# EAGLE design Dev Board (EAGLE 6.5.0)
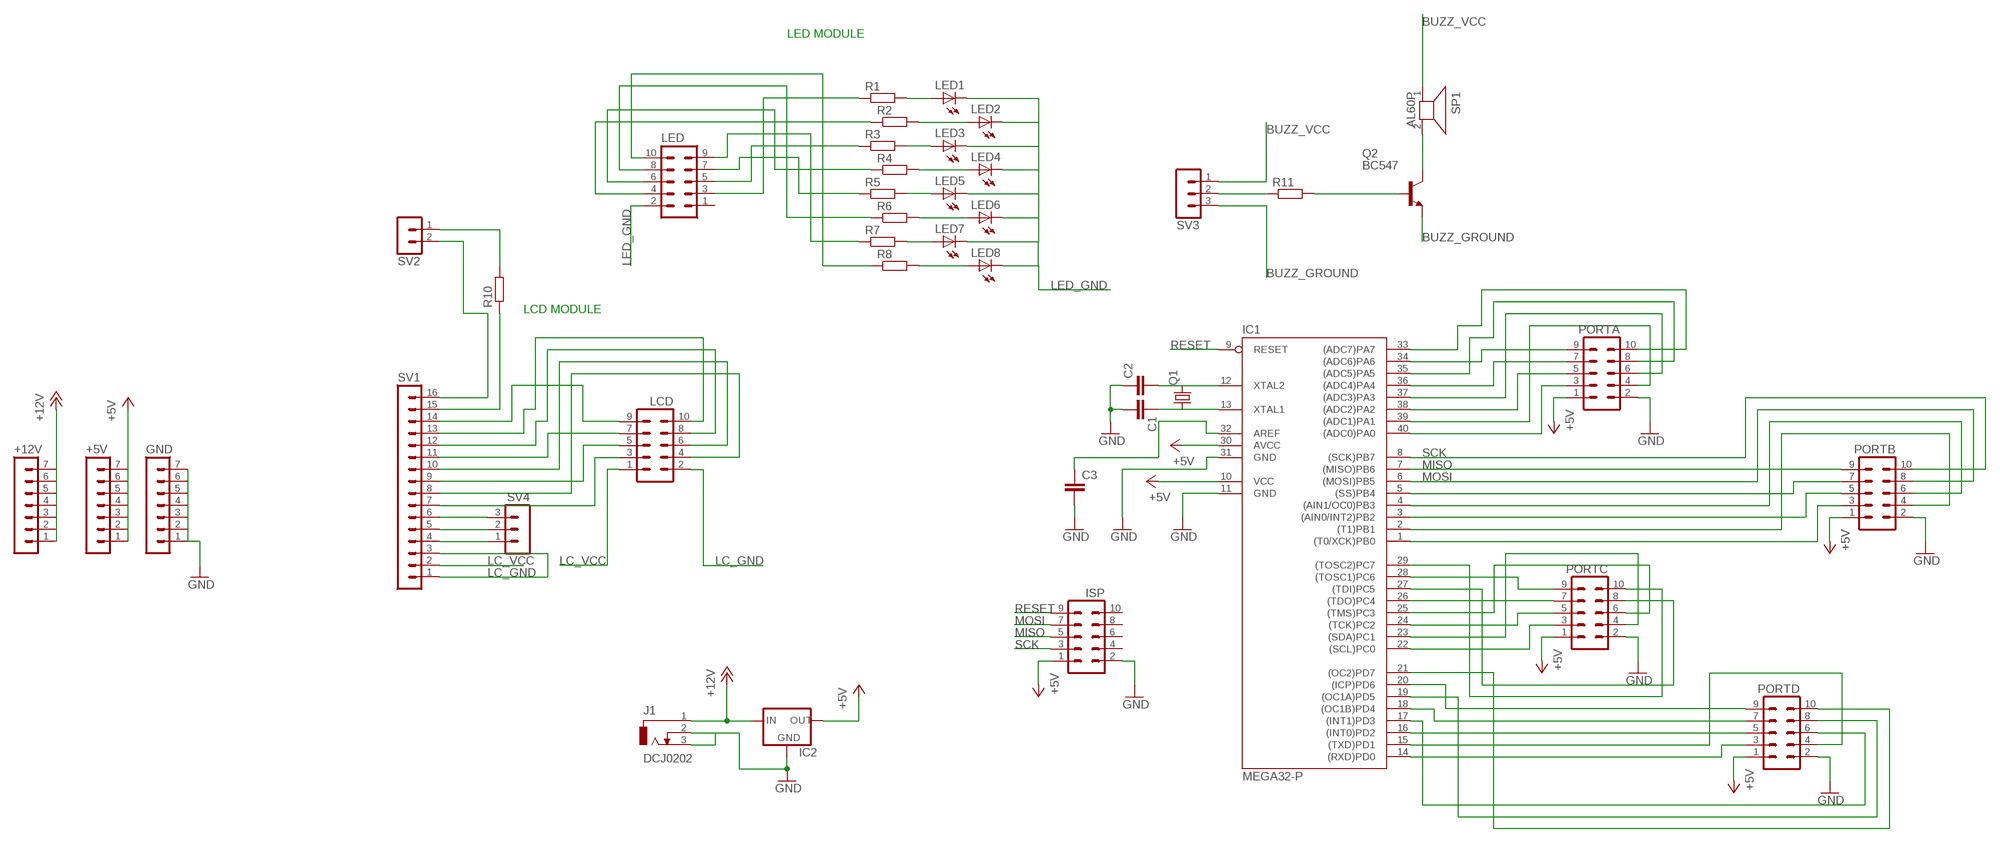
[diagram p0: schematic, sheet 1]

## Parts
+5V  MA07-1  [MA07-1]
+12V  MA07-1  [MA07-1]
C1  C-EU025-024X044  [C025-024X044]
C2  C-EU025-024X044  [C025-024X044]
C3  C-EU025-024X044  [C025-024X044]
GND  MA07-1  [MA07-1]
IC1  MEGA32-P  [DIL40]
IC2  78XXL  [78XXL]
ISP  MA05-2  [MA05-2]
J1  DCJ0202  [DCJ0202]
LCD  MA05-2  [MA05-2]
LED  MA05-2  [MA05-2]
LED1  LED3MM  [LED3MM]
LED2  LED3MM  [LED3MM]
LED3  LED3MM  [LED3MM]
LED4  LED3MM  [LED3MM]
LED5  LED3MM  [LED3MM]
LED6  LED3MM  [LED3MM]
LED7  LED3MM  [LED3MM]
LED8  LED3MM  [LED3MM]
PORTA  MA05-2  [MA05-2]
PORTB  MA05-2  [MA05-2]
PORTC  MA05-2  [MA05-2]
PORTD  MA05-2  [MA05-2]
Q1  CRYSTALHC49S  [HC49/S]
Q2  BC547  [TO92]
R1  R-EU_0207/10  [0207/10]
R2  R-EU_0207/10  [0207/10]
R3  R-EU_0207/10  [0207/10]
R4  R-EU_0207/10  [0207/10]
R5  R-EU_0207/10  [0207/10]
R6  R-EU_0207/10  [0207/10]
R7  R-EU_0207/10  [0207/10]
R8  R-EU_0207/10  [0207/10]
R10  R-EU_0207/10  [0207/10]
R11  R-EU_0207/10  [0207/10]
SP1  AL60P  [AL60P]
SV1  MA13-1  [MA13-1]
SV2  MA03-1  [MA03-1]
SV3  MA03-1  [MA03-1]
SV4  MA03-1  [MA03-1]

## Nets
+5V: +5V.1 +5V.2 +5V.3 +5V.4 +5V.5 +5V.6 +5V.7 IC1.10(VCC) IC1.30(AVCC) IC2.OUT ISP.1 PORTA.1 PORTB.1 PORTC.1 PORTD.1
+12V: +12V.1 +12V.2 +12V.3 +12V.4 +12V.5 +12V.6 +12V.7 IC2.IN J1.1
BUZZ_GROUND: Q2.1(E) SV3.3
BUZZ_VCC: SP1.1 SV3.1
GND: C1.2 C2.1 C3.2 GND.1 GND.2 GND.3 GND.4 GND.5 GND.6 GND.7 IC1.11(GND) IC1.31(GND) IC2.GND ISP.2 J1.2 J1.3 PORTA.2 PORTB.2 PORTC.2 PORTD.2
LC_GND: LCD.2 SV1.1 SV1.3
LC_VCC: LCD.1 SV1.2
LCD_GND: SV1.16 SV2.2
LED_GND: LED1.K(C) LED2.K(C) LED3.K(C) LED4.K(C) LED5.K(C) LED6.K(C) LED7.K(C) LED8.K(C) LED.2
MISO: IC1.7((MISO)PB6) ISP.5 PORTB.9
MOSI: IC1.6((MOSI)PB5) ISP.7 PORTB.8
N$1: LED1.A R1.2
N$2: LED2.A R2.2
N$3: LED3.A R3.2
N$4: LED4.A R4.2
N$5: LED5.A R5.2
N$6: LED6.A R6.2
N$7: LED7.A R7.2
N$8: LED8.A R8.2
N$9: IC1.40((ADC0)PA0) PORTA.3
N$10: IC1.38((ADC2)PA2) PORTA.5
N$11: IC1.36((ADC4)PA4) PORTA.7
N$12: IC1.34((ADC6)PA6) PORTA.9
N$13: IC1.39((ADC1)PA1) PORTA.4
N$14: IC1.37((ADC3)PA3) PORTA.6
N$15: IC1.35((ADC5)PA5) PORTA.8
N$17: LED.3 R1.1
N$18: LED.4 R2.1
N$19: LED.5 R3.1
N$20: LED.6 R4.1
N$21: LED.7 R5.1
N$22: LED.8 R6.1
N$23: LED.9 R7.1
N$24: LED.10 R8.1
N$25: IC1.33((ADC7)PA7) PORTA.10
N$26: IC1.1((T0/XCK)PB0) PORTB.3
N$27: IC1.3((AIN0/INT2)PB2) PORTB.5
N$28: IC1.5((SS)PB4) PORTB.7
N$30: IC1.2((T1)PB1) PORTB.4
N$31: IC1.4((AIN1/OC0)PB3) PORTB.6
N$32: R10.1 SV1.15
N$33: Q2.2(B) R11.2
N$34: IC1.22((SCL)PC0) PORTC.3
N$35: IC1.24((TCK)PC2) PORTC.5
N$36: IC1.26((TDO)PC4) PORTC.7
N$37: IC1.28((TOSC1)PC6) PORTC.9
N$38: IC1.23((SDA)PC1) PORTC.4
N$39: IC1.25((TMS)PC3) PORTC.6
N$40: IC1.27((TDI)PC5) PORTC.8
N$41: IC1.29((TOSC2)PC7) PORTC.10
N$42: IC1.14((RXD)PD0) PORTD.3
N$43: IC1.16((INT0)PD2) PORTD.5
N$44: IC1.18((OC1B)PD4) PORTD.7
N$45: IC1.20((ICP)PD6) PORTD.9
N$46: IC1.15((TXD)PD1) PORTD.4
N$47: IC1.17((INT1)PD3) PORTD.6
N$48: IC1.19((OC1A)PD5) PORTD.8
N$49: IC1.21((OC2)PD7) PORTD.10
N$50: C2.2 IC1.12(XTAL2) Q1.2
N$51: C1.1 IC1.13(XTAL1) Q1.1
N$52: SV1.4 SV4.1
N$53: LCD.3 SV1.7
N$54: SV1.5 SV4.2
N$55: SV1.6 SV4.3
N$56: LCD.5 SV1.9
N$57: LCD.7 SV1.11
N$58: LCD.9 SV1.14
N$59: LCD.4 SV1.8
N$60: LCD.6 SV1.10
N$61: LCD.8 SV1.12
N$62: LCD.10 SV1.13
N$63: R10.2 SV2.1
N$64: C3.1 IC1.32(AREF)
N$65: Q2.3(C) SP1.2
N$68: R11.1 SV3.2
RESET: IC1.9(RESET) ISP.9
SCK: IC1.8((SCK)PB7) ISP.3 PORTB.10
Unconnected: ISP.4 ISP.6 ISP.8 ISP.10 LED.1

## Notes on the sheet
- LED MODULE
- LCD MODULE

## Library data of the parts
+5V +12V GND = con-lstb:MA07-1: PIN HEADER; OC_FARNELL: unknown; OC_NEWARK: unknown
C1-C3 = rcl:C-EU: CAPACITOR, European symbol
IC1 = atmel:MEGA32-P: MICROCONTROLLER 32 Kbytes FLASH 2 Kbytes SRAM 1 Kbytes EEPROM USART 8-channel 10 bit ADC Source: www.atmel.com .. doc2503.pdf; MPN: ATMEGA32-16PU; OC_FARNELL: 1661729; OC_NEWARK: 51P1794
IC2 = v-reg:78XXL: VOLTAGE REGULATOR
ISP LCD LED PORTA PORTB PORTC PORTD = con-lstb:MA05-2: PIN HEADER; OC_FARNELL: unknown; OC_NEWARK: unknown
J1 = con-jack:DCJ0202: DC POWER JACK Source: DCJ0202.pdf; OC_FARNELL: unknown; OC_NEWARK: unknown
LED1-LED8 = led:LED: LED
Q1 = crystal:CRYSTAL: CRYSTAL; OC_FARNELL: 1667008; OC_NEWARK: unknown
Q2 = transistor-npn:BC547*: NPN Transistor
R1-R8 R10 R11 = rcl:R-EU_: RESISTOR, European symbol
SP1 = buzzer:AL60P: SPEAKER; OC_FARNELL: unknown; OC_NEWARK: unknown
SV1 = con-lstb-modified:MA13-1: PIN HEADER; OC_FARNELL: unknown; OC_NEWARK: unknown
SV2 = con-lstb-modified:MA03-1: PIN HEADER; OC_FARNELL: unknown; OC_NEWARK: unknown
SV3 SV4 = con-lstb:MA03-1: PIN HEADER; OC_FARNELL: unknown; OC_NEWARK: unknown

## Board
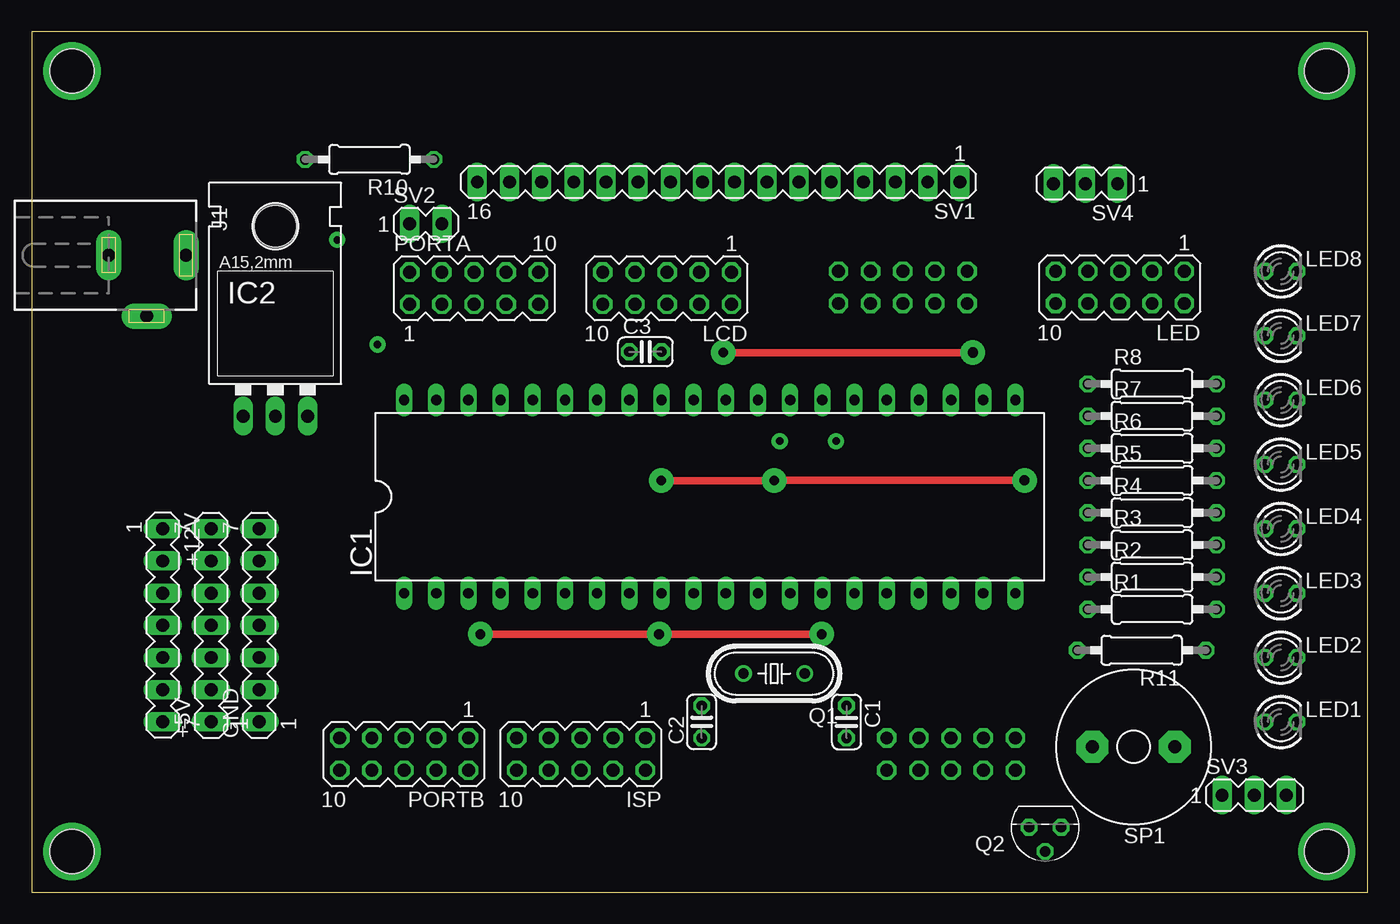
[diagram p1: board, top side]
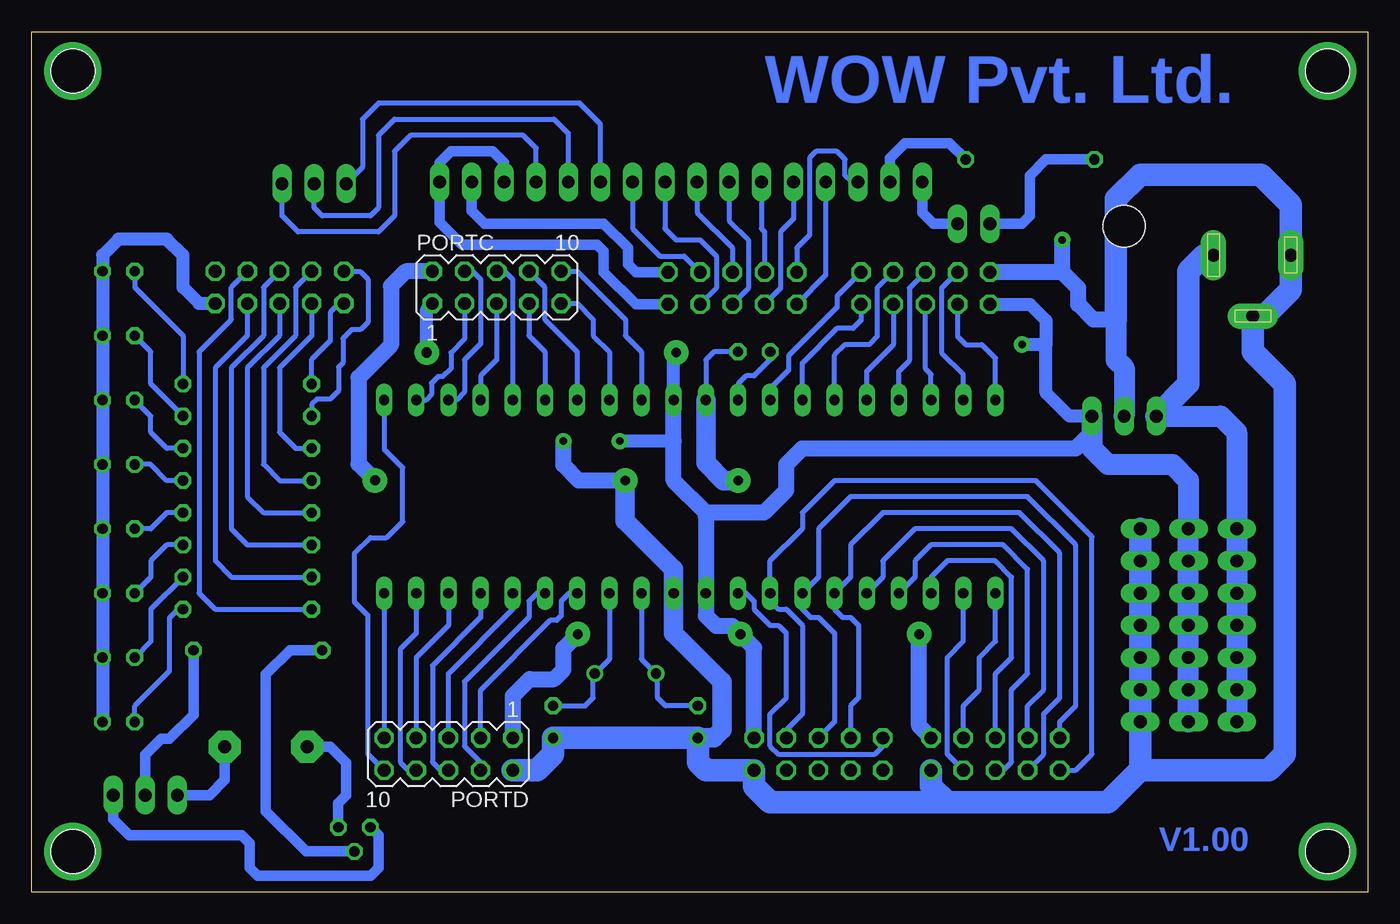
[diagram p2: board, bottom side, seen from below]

Size 105.48 x 67.9 mm. Coordinates in mm from the lower left corner, seen from the top.
Outline: 0,0 105.48,0 105.48,67.9 0,67.9 0,0
Copper layers (1*16): Top 0.035mm / dielectric 1.5mm / Bottom 0.035mm
Design rules "default": minimum track width 10mil, minimum drill 24mil, track to track 8mil, track to pad 8mil, pad to pad 8mil, via to via 8mil, smd to smd 8mil, copper to edge 40mil, drill to drill 8mil, minimum pad ring 10mil, minimum via ring 8mil, stop-mask expansion 4mil, vias tented up to drill 0mil, thermal gap 10mil
Holes 3.5 mm at 3.17,64.8 3.17,3.21 102.23,3.21 102.23,64.8

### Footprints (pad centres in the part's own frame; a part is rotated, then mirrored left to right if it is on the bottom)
MA07-1 = drill 1.016 long: 1 -7.62,0; 2 -5.08,0; 3 -2.54,0; 4 0,0; 5 2.54,0; 6 5.08,0; 7 7.62,0
C025-024X044 = drill 0.813 octagon: 1 -1.27,0; 2 1.27,0
DIL40 = drill 0.813 long: 1 -24.13,-7.62; 2 -21.59,-7.62; 3 -19.05,-7.62; 4 -16.51,-7.62; 5 -13.97,-7.62; 6 -11.43,-7.62; 7 -8.89,-7.62; 8 -6.35,-7.62; 9 -3.81,-7.62; 10 -1.27,-7.62; 11 1.27,-7.62; 12 3.81,-7.62; 13 6.35,-7.62; 14 8.89,-7.62; 15 11.43,-7.62; 16 13.97,-7.62; 17 16.51,-7.62; 18 19.05,-7.62; 19 21.59,-7.62; 20 24.13,-7.62; 21 24.13,7.62; 22 21.59,7.62; 23 19.05,7.62; 24 16.51,7.62; 25 13.97,7.62; 26 11.43,7.62; 27 8.89,7.62; 28 6.35,7.62; 29 3.81,7.62; 30 1.27,7.62; 31 -1.27,7.62; 32 -3.81,7.62; 33 -6.35,7.62; 34 -8.89,7.62; 35 -11.43,7.62; 36 -13.97,7.62; 37 -16.51,7.62; 38 -19.05,7.62; 39 -21.59,7.62; 40 -24.13,7.62
78XXL = drill 1.016 long: GND 0,-3.81; IN -2.54,-3.81; OUT 2.54,-3.81 | hole 3.302: 0,11.176
MA05-2 = drill 1.016 octagon: 1 -5.08,-1.27; 2 -5.08,1.27; 3 -2.54,-1.27; 4 -2.54,1.27; 5 0,-1.27; 6 0,1.27; 7 2.54,-1.27; 8 2.54,1.27; 9 5.08,-1.27; 10 5.08,1.27
DCJ0202 = drill 1 pad 2 long: 1 0,3.1; 2 4.8,0; 3 0,-3
LED3MM = drill 0.813 octagon: A -1.27,0; K 1.27,0
HC49/S = drill 0.813: 1 -2.413,0; 2 2.413,0
TO92 = drill 0.813 octagon: 1 1.27,0; 2 0,1.905; 3 -1.27,0
0207/10 = drill 0.813 octagon: 1 -5.08,0; 2 5.08,0
AL60P = drill 1.016 pad 2.54 octagon: 1 -3.251,0; 2 3.251,0
MA13-1 = drill 1.016 long: 1 -19.05,0; 2 -16.51,0; 3 -13.97,0; 4 -11.43,0; 5 -8.89,0; 6 -6.35,0; 7 -3.81,0; 8 -1.27,0; 9 1.27,0; 10 3.81,0; 11 6.35,0; 12 8.89,0; 13 11.43,0; 14 13.97,0; 15 16.51,0; 16 19.05,0
MA03-1 = drill 1.016 long: 1 -2.54,0; 2 0,0
MA03-1' = drill 1.016 long: 1 -2.54,0; 2 0,0; 3 2.54,0

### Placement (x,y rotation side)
+5V  14.16,21.05 90 top
+12V  10.35,21.05 270 top
C1  64.33,13.43 270 top
C2  52.9,13.43 90 top
C3  48.45,42.64 0 top
GND  17.97,21.05 90 top
IC1  53.53,31.21 0 top
IC2  19.24,41.37 0 top
ISP  43.37,10.89 180 top
J1  9.08,50.26 270 top
LCD  50.16,47.66 180 top
LED  85.92,47.72 180 top
LED1  98.61,13.43 0 top
LED2  98.61,18.51 0 top
LED3  98.61,23.59 0 top
LED4  98.61,28.67 0 top
LED5  98.61,33.75 0 top
LED6  98.61,38.83 0 top
LED7  98.61,43.91 0 top
LED8  98.61,48.99 0 top
PORTA  34.92,47.66 0 top
PORTB  29.4,10.89 180 top
PORTC  68.77,47.72 0 bottom
PORTD  72.58,10.89 180 bottom
Q1  58.61,17.24 180 top
Q2  80.01,5.11 180 top
R1  88.45,22.32 0 top
R2  88.45,24.86 0 top
R3  88.45,27.4 0 top
R4  88.45,29.94 0 top
R5  88.45,32.48 0 top
R6  88.45,35.02 0 top
R7  88.45,37.56 0 top
R8  88.45,40.1 0 top
R10  26.67,57.82 180 top
R11  87.63,19.08 180 top
SP1  87,11.46 180 top
SV1  54.23,56.04 180 top
SV2  32.38,52.74 0 top
SV3  [MA03-1']  96.52,7.65 0 top
SV4  [MA03-1']  83.19,55.91 180 top

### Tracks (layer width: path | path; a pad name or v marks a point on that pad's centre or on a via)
+5V  (via drill 0.6 pad 1.27, 0.76 pad 1.93, 0.8 pad 1.93)
  Top 0.61: v62.36,20.35 v49.53,20.35 v35.43,20.35 | v54.61,42.58 v74.3,42.58
  Bottom 1.016: IC2.OUT 23.56,37.56 25.4,39.4 25.4,43.21 | PORTA.1 26.67,46.39 25.4,45.12 25.4,43.21 | v74.3,42.58 74.3,46 PORTC.1 | IC1.30 54.8,42.39 v54.61,42.58 | 25.4,43.21 v27.3,43.21 | 54.8,35.59 v59.05,35.59
  Bottom 1.27: PORTD.1 67.5,15.46 66.17,16.8 64.26,16.8 63.5,17.56 63.5,19.21 v62.36,20.35 | +5V.1 +5V.7 | IC2.OUT 21.78,36.29 23.05,35.02 44.64,35.02 45.91,33.75 45.91,31.72 47.69,29.94 52.01,29.94 52.26,29.69 | 52.26,29.69 52.26,29.94 54.8,32.48 54.8,35.59 IC1.30 | 52.26,29.69 IC1.10 52.26,21.81 51.44,20.99 50.16,20.99 v49.53,20.35 48.45,19.27 ISP.1 | PORTB.1 35.43,13.11 v35.43,20.35
  Bottom 1.676: +5V.1 +5V.2 +5V.3 +5V.4 +5V.5 +5V.6 +5V.7 14.16,32.48 15.43,33.75 20.51,33.75 21.78,35.02 IC2.OUT
+12V
  Bottom 1.676: +12V.7 +12V.6 +12V.5 +12V.4 +12V.3 +12V.2 +12V.1 10.35,36.29 11.62,37.56 IC2.IN
  Bottom 1.778: J1.1 12.89,50.26 14.16,48.99 14.16,40.1 IC2.IN
BUZZ_GROUND
  Bottom 0.813: SV3.3 99.06,5.75 97.79,4.48 88.9,4.48 88.27,3.84 88.27,1.94 87.63,1.3 78.74,1.3 78.11,1.94 78.11,4.48 Q2.1
BUZZ_VCC
  Bottom 0.813: SP1.1 90.25,8.85 91.44,7.65 SV3.1
GND  (via drill 0.6 pad 1.27, 0.6 pad 1.78, 0.76 pad 1.93, 0.8 pad 1.93)
  Top 0.61: v58.61,32.48 v49.72,32.48 v49.71,32.47 | v58.62,32.49 v78.38,32.49
  Top 1.27: v58.62,32.49 v58.61,32.48
  Bottom 0.406: C3.2 51.62,42.64 52.26,42 IC1.31
  Bottom 1.27: 19.88,45.18 21.65,45.18 22.86,46.39 22.86,47.66 24.13,48.93 | 24.13,48.93 PORTA.2 | PORTC.2 75.96,48.99 77.11,47.83 77.11,43.16 79.68,40.6 79.68,33.79 v78.38,32.49 | v58.61,32.48 62.29,32.48 63.5,33.69 v63.5,35.59 | 24.13,48.93 v24.13,51.47
  Bottom 1.524: C2.1 51.62,12.16 50.99,12.79 50.99,16.61 54.8,20.41 IC1.11 54.8,25.5 58.62,29.32 v58.62,32.49 | v49.71,32.47 50.85,32.47 52.26,33.88 IC1.31
  Bottom 1.676: 19.88,45.18 19.88,42 19.24,41.37 IC2.GND
  Bottom 1.778: GND.7 GND.6 GND.5 GND.4 GND.3 GND.2 GND.1 17.97,9.62 | 33.21,7.08 34.48,8.35 PORTB.2 | 33.21,7.08 47.18,7.08 48.45,8.35 ISP.2 52.26,9.62 52.9,10.26 C2.1 C1.2 64.33,10.89 65.59,9.62 PORTD.2 | 19.88,45.18 19.88,54.7 17.97,56.61 8.45,56.61 6.08,54.24 J1.3 6.08,47.54 8.16,45.46 J1.2 9.08,42.64 6.54,40.1 6.54,10.89 7.81,9.62 17.97,9.62 | 33.21,7.08 20.51,7.08 18.22,9.37 17.97,9.62
LC_GND
  Bottom 0.813: LCD.2 57.78,46.39 60.33,48.93 60.33,50.58 60.83,51.09 71.5,51.09 73.28,52.86 SV1.1 73.28,57.56 72.39,58.45 69.09,58.45 68.2,57.56 SV1.3
LC_VCC
  Bottom 0.813: SV1.2 70.74,53.75 69.72,52.74 60.33,52.74 58.42,50.83 58.42,49.56 57.78,48.93 LCD.1
LCD_GND
  Bottom 0.813: SV1.16 35.18,53.63 34.29,52.74 SV2.2
LED_GND
  Bottom 1.016: LED1.K LED2.K LED3.K LED4.K LED5.K LED6.K LED7.K LED8.K 99.89,50.26 98.61,51.53 94.81,51.53 93.53,50.26 93.53,47.72 92.27,46.45 LED.2
MISO
  Bottom 0.406: ISP.5 42.1,13.43 42.1,20.41 43.37,21.68 44.01,21.68 44.64,22.32 IC1.7 43.37,24.86 43.37,28.67 40.83,31.21 26.86,31.21 23.05,27.4 23.05,14.7 24.32,13.43 PORTB.9
MOSI
  Bottom 0.406: ISP.7 40.83,14.7 40.2,15.34 40.2,21.05 40.83,21.68 41.47,21.68 42.1,22.32 IC1.6 40.83,24.86 40.83,27.4 38.29,29.94 27.5,29.94 24.32,26.77 24.32,15.34 25.59,14.06 25.59,10.89 PORTB.8
N$1
  Bottom 0.406: LED1.A 97.34,14.7 94.61,17.43 94.61,21.62 93.92,22.32 R1.2
N$2
  Bottom 0.406: R2.2 96.08,22.32 96.08,19.78 LED2.A
N$3
  Bottom 0.406: R3.2 94.81,27.4 96.08,26.13 96.08,24.86 LED3.A
N$4
  Bottom 0.406: R4.2 94.81,29.94 96.08,28.67 LED4.A
N$5
  Bottom 0.406: R5.2 94.81,32.48 96.08,33.75 LED5.A
N$6
  Bottom 0.406: R6.2 94.81,35.02 96.08,36.29 96.08,37.56 LED6.A
N$7
  Bottom 0.406: R7.2 96.08,40.1 96.08,42.64 LED7.A
N$8
  Bottom 0.406: LED8.A 97.34,47.72 93.53,43.91 R8.2
N$9
  Bottom 0.406: PORTA.3 32.38,43.85 31.75,43.21 30.48,43.21 29.4,42.13 IC1.40
N$10
  Bottom 0.406: IC1.38 34.48,40.86 34.92,41.31 PORTA.5
N$11
  Bottom 0.406: PORTA.7 37.47,43.21 39.56,41.12 IC1.36
N$12
  Bottom 0.406: PORTA.9 40.01,45.12 40.64,44.48 41.91,44.48 44.64,41.75 IC1.34
N$13
  Bottom 0.406: PORTA.4 33.66,47.66 33.66,42.58 31.94,40.86 IC1.39
N$14
  Bottom 0.406: IC1.37 37.02,41.12 36.2,41.94 36.2,47.66 PORTA.6
N$15
  Bottom 0.406: PORTA.8 38.73,47.66 38.73,43.85 39.37,43.21 41.27,43.21 42.1,42.39 IC1.35
N$16  (via drill 3.5 pad 0.3)
  other vias: 3.17,64.8
N$17
  Bottom 0.406: LED.3 89.72,47.72 89.72,45.18 92.27,42.64 92.27,23.59 91,22.32 R1.1
N$18
  Bottom 0.406: R2.1 89.72,24.86 91,26.13 91,41.37 88.45,43.91 LED.4
N$19
  Bottom 0.406: LED.5 87.19,47.72 87.19,43.91 89.72,41.37 89.72,28.67 88.45,27.4 R3.1
N$20
  Bottom 0.406: LED.6 85.92,43.91 88.45,41.37 88.45,31.21 87.19,29.94 R4.1
N$21
  Bottom 0.406: LED.7 84.64,47.72 84.64,43.91 87.19,41.37 87.19,33.75 85.92,32.48 R5.1
N$22
  Bottom 0.406: LED.8 83.38,43.91 85.92,41.37 85.92,36.29 84.64,35.02 R6.1
N$23
  Bottom 0.406: LED.9 79.56,48.99 78.93,48.35 78.93,44.98 79.53,44.38 80.21,44.38 80.9,43.69 80.9,41.79 81.25,41.43 81.25,39.55 81.92,38.89 82.96,38.89 83.36,38.49 83.36,37.57 R7.1
N$24
  Bottom 0.406: LED.10 81.22,46.45 81.92,45.75 81.92,43.49 83.38,42.03 R8.1
N$25
  Bottom 0.406: PORTA.10 41.91,47.02 41.91,46.13 45.72,42.32 45.72,41.18 47.18,39.72 IC1.33
N$26
  Bottom 0.406: PORTB.3 31.94,14.7 30.67,15.97 30.67,18.51 29.4,19.78 IC1.1
N$27
  Bottom 0.406: PORTB.5 29.4,17.24 28.13,18.51 28.13,24.86 29.4,26.13 33.21,26.13 34.48,24.86 IC1.3
N$28
  Bottom 0.406: PORTB.7 26.86,14.7 25.59,15.97 25.59,26.13 28.13,28.67 35.75,28.67 38.29,26.13 38.29,24.86 IC1.5
N$30
  Bottom 0.406: PORTB.4 33.21,10.89 33.21,18.51 31.94,19.78 IC1.2
N$31
  Bottom 0.406: PORTB.6 28.77,9.62 28.13,10.26 28.13,15.97 26.86,17.24 26.86,25.5 28.77,27.4 34.48,27.4 35.75,26.13 35.75,24.86 IC1.4
N$32
  Bottom 0.813: R10.1 33.02,59.09 36.55,59.09 37.72,57.92 SV1.15
N$33
  Bottom 0.813: R11.2 85.09,19.08 87,17.18 87,6.38 83.82,3.21 Q2.2
N$34
  Bottom 0.406: PORTC.3 71.31,43.66 72.39,42.58 72.39,41.31 73.03,40.67 73.41,40.67 73.91,40.16 73.91,39.27 74.36,38.83 IC1.22
N$35
  Bottom 0.406: PORTC.5 68.77,42 70.04,40.73 IC1.24
N$36
  Bottom 0.406: PORTC.7 66.23,43.91 64.96,42.64 IC1.26
N$37
  Bottom 0.406: PORTC.9 62.42,46.45 61.15,45.18 61.15,43.91 59.88,42.64 IC1.28
N$38
  Bottom 0.406: PORTC.4 70.67,48.99 70.04,48.35 70.04,43.27 71.31,42 71.31,39.46 71.94,38.83 IC1.23
N$39
  Bottom 0.406: PORTC.6 68.14,48.99 67.5,48.35 IC1.25
N$40
  Bottom 0.406: PORTC.8 64.96,47.72 64.96,45.18 62.42,42.64 IC1.27
N$41
  Bottom 0.406: PORTC.10 62.42,48.99 58.61,45.18 58.61,43.91 57.34,42.64 IC1.29
N$42
  Bottom 0.406: IC1.14 63.05,23.59 63.69,22.95 63.69,21.79 64.03,21.44 64.54,21.44 70.04,15.95 PORTD.3
N$43
  Bottom 0.406: PORTD.5 72.58,17.24 67.5,22.32 IC1.16
N$44
  Bottom 0.406: IC1.18 72.58,21.05 75.12,18.51 PORTD.7
N$45
  Bottom 0.406: IC1.20 PORTD.9
N$46
  Bottom 0.406: PORTD.4 70.04,10.26 71.31,11.53 71.31,16.61 66.23,21.68 66.23,22.95 65.59,23.59 IC1.15
N$47
  Bottom 0.406: IC1.17 70.04,21.68 73.85,17.88 73.85,10.26 73.22,9.62 PORTD.6
N$48
  Bottom 0.406: IC1.19 75.12,20.41 76.39,19.14 76.39,10.26 75.75,9.62 PORTD.8
N$49
  Bottom 0.406: PORTD.10 78.93,10.89 78.93,21.81 80.01,22.89 80.01,26.7 78.74,27.97 77.47,27.97 76.2,29.24 76.2,33.5 77.66,34.96 IC1.21
N$50
  Bottom 0.406: IC1.12 57.34,18.38 Q1.2 56.07,17.11 56.07,15.34 55.44,14.7 C2.2
N$51
  Bottom 0.406: IC1.13 59.88,18.38 Q1.1 61.15,17.11 61.15,15.34 61.78,14.7 C1.1
N$52
  Bottom 0.406: SV1.4 65.66,58.71 66.67,59.72 75.56,59.72 76.83,58.45 76.83,53.37 78.11,52.1 84.45,52.1 85.72,53.37 SV4.1
N$53
  Bottom 0.406: SV1.7 58.04,52.36 55.88,50.2 53.98,50.2 LCD.3
N$54
  Bottom 0.406: SV1.5 63.12,59.85 64.26,60.99 76.83,60.99 78.11,59.72 78.11,54.01 78.74,53.37 82.55,53.37 83.19,54.01 SV4.2
N$55
  Bottom 0.406: SV1.6 60.58,60.61 62.23,62.26 78.11,62.26 79.38,60.99 79.38,57.18 SV4.3
N$56
  Bottom 0.406: SV1.9 52.96,53.63 50.16,50.83 LCD.5
N$57
  Bottom 0.406: SV1.11 47.88,52.36 47.62,52.1 LCD.7
N$58
  Bottom 0.406: SV1.14 40.77,56.04 41.27,56.55 41.27,57.82 41.91,58.45 43.56,58.45 44.07,57.94 44.07,51.85 45.09,50.83 LCD.9
N$59
  Bottom 0.406: SV1.8 55.5,52.36 54.61,51.47 52.7,51.47 51.44,50.2 51.44,47.66 LCD.4
N$60
  Bottom 0.406: SV1.10 50.42,52.99 48.9,51.47 48.9,47.66 LCD.6
N$61
  Bottom 0.406: SV1.12 45.34,53.12 46.35,52.1 46.35,47.66 LCD.8
N$62
  Bottom 0.406: SV1.13 42.8,48.67 LCD.10
N$63
  Bottom 0.813: R10.2 25.4,57.82 26.67,56.55 26.67,53.37 27.3,52.74 SV2.1
N$64
  Bottom 0.406: C3.1 47.18,42 48.45,40.73 49.09,40.73 49.72,40.1 IC1.32
N$65
  Bottom 0.813: SP1.2 81.92,11.46 80.64,10.19 80.64,7.65 81.28,7.02 Q2.3
N$66  (via drill 3.5 pad 0.3)
  other vias: 3.17,3.21
N$67  (via drill 3.5 pad 0.3)
  other vias: 102.23,3.21
N$68
  Bottom 0.813: R11.1 92.71,14 94.61,12.1 95.25,12.1 96.52,10.83 SV3.2
N$69  (via drill 3.5 pad 0.3)
  other vias: 102.23,64.8
RESET
  Bottom 0.406: ISP.9 38.29,11.53 38.92,10.89 46.55,10.89 47.18,11.53 47.18,14.06 45.91,15.34 45.91,20.41 46.55,21.05 47.18,21.05 48.45,22.32 48.45,22.95 49.09,23.59 IC1.9
SCK
  Bottom 0.406: ISP.3 45.91,12.79 44.64,14.06 44.64,21.05 45.91,22.32 46.55,22.32 47.18,22.95 IC1.8 47.18,26.13 44.64,28.67 44.64,29.94 42.1,32.48 26.23,32.48 21.78,28.04 21.78,10.89 23.05,9.62 PORTB.10

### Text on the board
Bottom: WOW Pvt. Ltd. | V1.00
